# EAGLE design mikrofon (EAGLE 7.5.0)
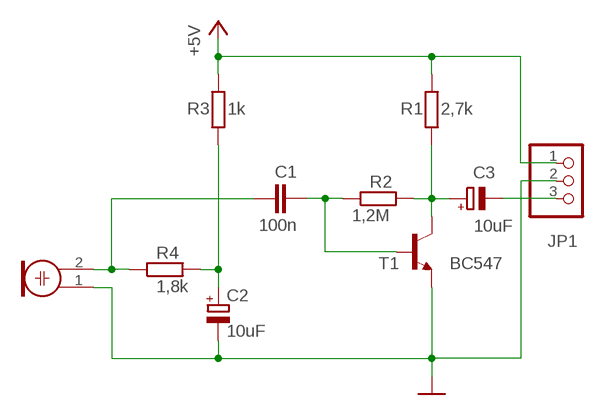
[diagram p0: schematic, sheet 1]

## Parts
C1  100n  C-EU025-025X050  [C025-025X050]
C2  10uF  CPOL-EUE2-4  [E2-4]
C3  10uF  CPOL-EUE2-4  [E2-4]
JP1  PINHD-1X3  [1X03]
M1  Mike  ELECTRET_MICROPHON-WM-61B  [WM-61B]
R1  2,7k  R-EU_0204/7  [0204/7]
R2  1,2M  R-EU_0204/7  [0204/7]
R3  1k  R-EU_0204/7  [0204/7]
R4  1,8k  R-EU_0204/7  [0204/7]
T1  BC547  BC547B-NPN-TO92-CBE  [TO92-CBE]

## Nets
+5V: JP1.1 R1.2 R3.2
GND: C2.- JP1.2 M1.1 T1.E
N$1: C1.1 M1.2 R4.1
N$2: C2.+ R3.1 R4.2
N$3: C1.2 R2.1 T1.B
N$4: C3.+ R1.1 R2.2 T1.C
N$6: C3.- JP1.3

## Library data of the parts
C1 = rcl:C-EU: CAPACITOR, European symbol
C2 C3 = rcl:CPOL-EU: POLARIZED CAPACITOR, European symbol
JP1 = pinhead:PINHD-1X3: PIN HEADER
M1 = microphon:ELECTRET_MICROPHON-: Electret Condenser Microphone
R1-R4 = rcl:R-EU_: RESISTOR, European symbol
T1 = transistor:*-NPN-: NPN Transistror BF959 corrected 2008.03.06

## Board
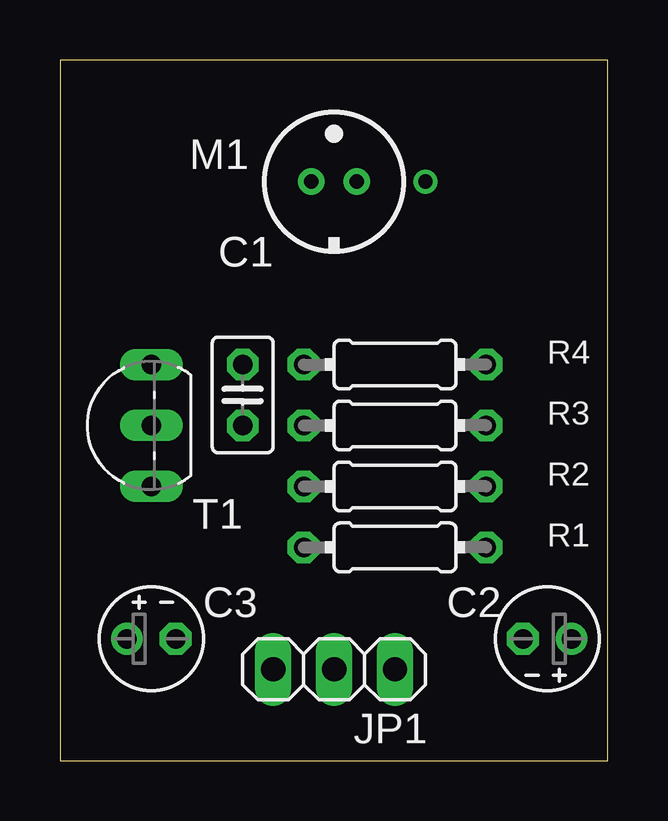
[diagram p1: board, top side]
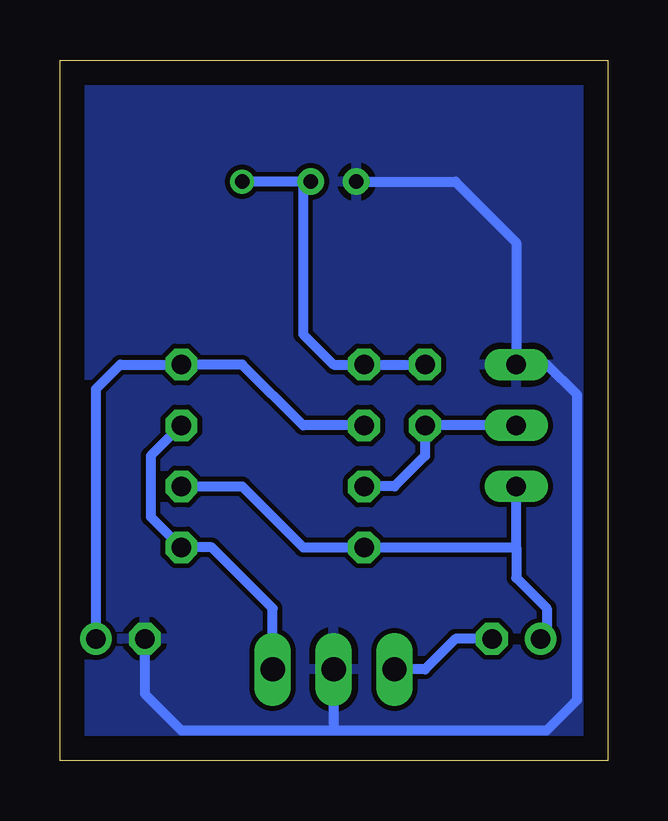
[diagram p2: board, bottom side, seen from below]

Size 22.84 x 29.2 mm. Coordinates in mm from the lower left corner, seen from the top.
Outline: 0,0 22.84,0 22.84,29.2 0,29.2 0,0
Copper layers (1*16): Top 0.035mm / dielectric 1.5mm / Bottom 0.035mm
Design rules "default": minimum track width 10mil, minimum drill 24mil, track to track 8mil, track to pad 8mil, pad to pad 8mil, via to via 8mil, smd to smd 8mil, copper to edge 40mil, drill to drill 8mil, minimum pad ring 10mil, minimum via ring 8mil, stop-mask expansion 4mil, vias tented up to drill 0mil, thermal gap 10mil

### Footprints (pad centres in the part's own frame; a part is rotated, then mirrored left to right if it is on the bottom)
C025-025X050 = drill 0.813 octagon: 1 -1.27,0; 2 1.27,0
E2-4 = drill 0.813 pad 1.27: + -1.016,0 | drill 0.813 pad 1.27 octagon: - 1.016,0
1X03 = drill 1.016 long: 1 -2.54,0; 2 0,0; 3 2.54,0
WM-61B = drill 0.6 pad 1: 1 0,0.95; 2 0,-0.95
0204/7 = drill 0.813 octagon: 1 -3.81,0; 2 3.81,0
TO92-CBE = drill 0.813 long: B 0,0; C -2.54,0; E 2.54,0

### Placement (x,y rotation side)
C1  7.62,15.24 270 top
C2  20.32,5.08 180 top
C3  3.81,5.08 0 top
JP1  11.43,3.81 180 top
M1  11.43,24.13 90 top
R1  13.97,8.89 0 top
R2  13.97,11.43 0 top
R3  13.97,13.97 0 top
R4  13.97,16.51 0 top
T1  3.81,13.97 90 top

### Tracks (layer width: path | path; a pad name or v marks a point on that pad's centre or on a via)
+5V
  Bottom 0.406: R3.2 19.05,12.7 19.05,10.16 R1.2 16.51,8.89 13.97,6.35 JP1.1
GND
  Bottom 0.406: M1.1 6.35,24.13 3.81,21.59 T1.E 2.54,16.51 1.27,15.24 1.27,2.54 2.54,1.27 11.43,1.27 | C2.- 19.3,2.79 17.78,1.27 11.43,1.27 | JP1.2 11.43,1.27
  pour Bottom: 0,29.21 22.86,29.21 22.86,0 0,0
N$1
  Bottom 0.406: M1.2 12.7,24.13 12.7,17.78 11.43,16.51 R4.1 C1.1
N$2
  Bottom 0.406: R3.1 12.7,13.97 15.24,16.51 R4.2 20.32,16.51 21.34,15.49 C2.+
N$3
  Bottom 0.406: T1.B C1.2 7.62,12.7 8.89,11.43 R2.1
N$4
  Bottom 0.406: 3.81,8.89 R1.1 12.7,8.89 15.24,11.43 R2.2 | 3.81,8.89 3.81,7.62 2.54,6.35 2.54,5.33 C3.+ | 3.81,8.89 T1.C
N$5  (via drill 0.6 pad 0.25)
  Bottom 0.406: 12.7,24.13 v15.24,24.13
N$6
  Bottom 0.406: C3.- 6.35,5.08 7.62,3.81 JP1.3

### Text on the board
tValues: +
